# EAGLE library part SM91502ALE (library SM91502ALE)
Surface Mount PCB Transformer Source: Datasheet
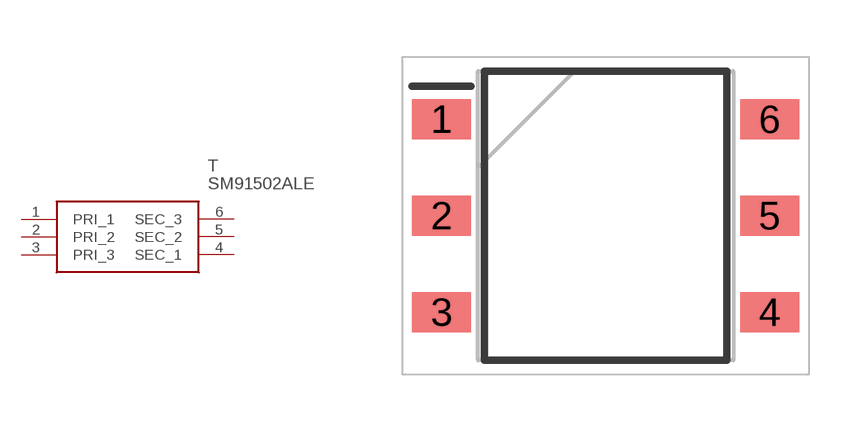
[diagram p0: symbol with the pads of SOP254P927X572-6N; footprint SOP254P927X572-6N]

Designator prefix T

## SM91502ALE (Description: Surface Mount PCB Transformer; Height: 5.72mm; Manufacturer_Name: Bourns; Manufacturer_Part_Number: SM91502ALE; Mouser_Part_Number: 652-SM91502ALE; Mouser_Price-Stock: https://www.mouser.co.uk/ProductDetail/Bourns/SM91502ALE?qs=qSfuJ%252Bfl%2Fd5OMMG8eLgKCQ%3D%3D)  [SOP254P927X572-6N]
1  PRI_1
2  PRI_2
3  PRI_3
4  SEC_1
5  SEC_2
6  SEC_3

## Footprint SOP254P927X572-6N (pad centres in mm)
SM9150
smd 1.55 x 1.05: 1 -4.325,2.54; 2 -4.325,0; 3 -4.325,-2.54; 4 4.325,-2.54; 5 4.325,0; 6 4.325,2.54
